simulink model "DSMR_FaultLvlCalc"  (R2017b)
settings: Solver=FixedStepDiscrete  StartTime=0.0  StopTime=10.0  FixedStep=0.02  RelTol=1e-3  EnableMultiTasking=on
undefined symbols (not defined in the file): bin2dec, BMS_DSMR_FaultLvlCalc, Delay, Delay1, DFES_Cls_DFC_638LinCommErr_C, DFES_Cls_DFC_AcDischgFobd_C, DFES_Cls_DFC_AChgFobd_C, DFES_Cls_DFC_AChgHVOffTmt_C, DFES_Cls_DFC_AChgHVOnTmt_C, DFES_Cls_DFC_AChgingErr_C, DFES_Cls_DFC_AChgLckTmt_C, DFES_Cls_DFC_AChgPileRdyTmt_C, DFES_Cls_DFC_AChgRdyPndiTmt_C, DFES_Cls_DFC_AChgRdyTmt_C, DFES_Cls_DFC_AChgS2ClsdTmt_C, DFES_Cls_DFC_AChgUnlckTmt_C, DFES_Cls_DFC_AChrgCnntErr_C, DFES_Cls_DFC_AChrgCurrMish_C, DFES_Cls_DFC_AChrgPortOvrTemp_C, DFES_Cls_DFC_AChrgVoltMish_C, DFES_Cls_DFC_AFEAdcRelatedErr_C, DFES_Cls_DFC_AFECellTempUpdErr_C, DFES_Cls_DFC_AFECellVoltLineOpen_C, DFES_Cls_DFC_AFECellVoltUpdErr_C, DFES_Cls_DFC_AFEComLost_C, DFES_Cls_DFC_AFEDiagModeExitErr_C, DFES_Cls_DFC_AFEGpioLineOpen_C, DFES_Cls_DFC_AFEOtherErr_C, DFES_Cls_DFC_AFEResetFlt_C, DFES_Cls_DFC_AFESampleErr_C, DFES_Cls_DFC_AFESplyFlt_C, DFES_Cls_DFC_AFETempHighFlt_C, DFES_Cls_DFC_APlusChk_C, DFES_Cls_DFC_BalCirOpenFlt_C, DFES_Cls_DFC_BalCirShortFlt_C, DFES_Cls_DFC_BalStuckMax_C, DFES_Cls_DFC_BalStuckMin_C, DFES_Cls_DFC_BalTempHighFlt_C, DFES_Cls_DFC_BattCurrMismatchErr_C, DFES_Cls_DFC_BattHVMsgTmt_C, DFES_Cls_DFC_BattSohChk_C, DFES_Cls_DFC_BattTAlrmMax_C, DFES_Cls_DFC_BattTAlrmMin_C, DFES_Cls_DFC_BattTCnstMax_C, DFES_Cls_DFC_BattTempVldMax_C, DFES_Cls_DFC_BattTempVldMin_C, DFES_Cls_DFC_BattTFaultMax_C, DFES_Cls_DFC_BattTFaultMin_C, DFES_Cls_DFC_BattTGradtMax_C, DFES_Cls_DFC_BattTHopMax_C, DFES_Cls_DFC_BattTWarnMax_C, DFES_Cls_DFC_BattTWarnMin_C, DFES_Cls_DFC_BattUNpl_C, DFES_Cls_DFC_BattVoltHiMax_C, DFES_Cls_DFC_BattVoltLoMin_C, DFES_Cls_DFC_BattVoltRngErr_C, DFES_Cls_DFC_BattVoltVld_C, DFES_Cls_DFC_BMSSplyPwrAbnToCAB_C, DFES_Cls_DFC_BMSSplyPwrAbnToLem_C, DFES_Cls_DFC_BoardTempTmt_C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
libraries: simulink x535
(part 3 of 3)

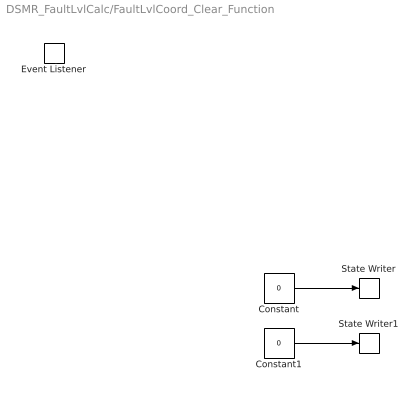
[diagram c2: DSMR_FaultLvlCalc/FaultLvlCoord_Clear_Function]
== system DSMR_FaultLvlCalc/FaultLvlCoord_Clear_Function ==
  Constant : Constant  Value=0  OutDataTypeStr=boolean
  Constant1 : Constant  Value=0  OutDataTypeStr=uint8
  Event Listener : EventListener  EventType=Reset  EventName=Clear  VariantControl=Variant
  State Writer : StateWriter  StateOwnerBlock=../../BMS_DSMR_FaultLvlCalc/FaultLvlCoord/Unit Delay
  State Writer1 : StateWriter  StateOwnerBlock=../../BMS_DSMR_FaultLvlCalc/FaultLvlCoord/Unit Delay1
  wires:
  Constant/1 -> State Writer/1
  Constant1/1 -> State Writer1/1

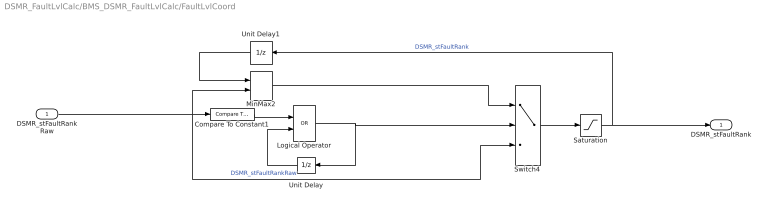
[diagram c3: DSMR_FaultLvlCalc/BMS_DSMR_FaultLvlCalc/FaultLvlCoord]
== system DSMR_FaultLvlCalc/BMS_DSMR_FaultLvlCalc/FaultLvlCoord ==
  DSMR_stFaultRankRaw : Inport
  Compare To Constant1 : simulink/Logic and Bit Operations/Compare To Constant  relop=>=  const=3  OutDataTypeStr=boolean
  Logical Operator : Logic  Operator=OR  AllPortsSameDT=off  OutDataTypeStr=boolean
  MinMax2 : MinMax  Function=max  Inputs=2
  Saturation : Saturate  UpperLimit=4  LowerLimit=0  OutDataTypeStr=uint8
  Switch4 : Switch  Criteria=u2 ~= 0
  Unit Delay : UnitDelay  SampleTime=-1
  Unit Delay1 : UnitDelay  SampleTime=-1
  DSMR_stFaultRank : Outport
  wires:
  MinMax2/1 -> Switch4/1
  Saturation/1 -> Unit Delay1/1, DSMR_stFaultRank/1  "DSMR_stFaultRank"
  DSMR_stFaultRankRaw/1 -> Switch4/3, Compare To Constant1/1, MinMax2/2  "DSMR_stFaultRankRaw"
  Switch4/1 -> Saturation/1
  Logical Operator/1 -> Switch4/2, Unit Delay/1
  Unit Delay1/1 -> MinMax2/1
  Compare To Constant1/1 -> Logical Operator/1
  Unit Delay/1 -> Logical Operator/2
